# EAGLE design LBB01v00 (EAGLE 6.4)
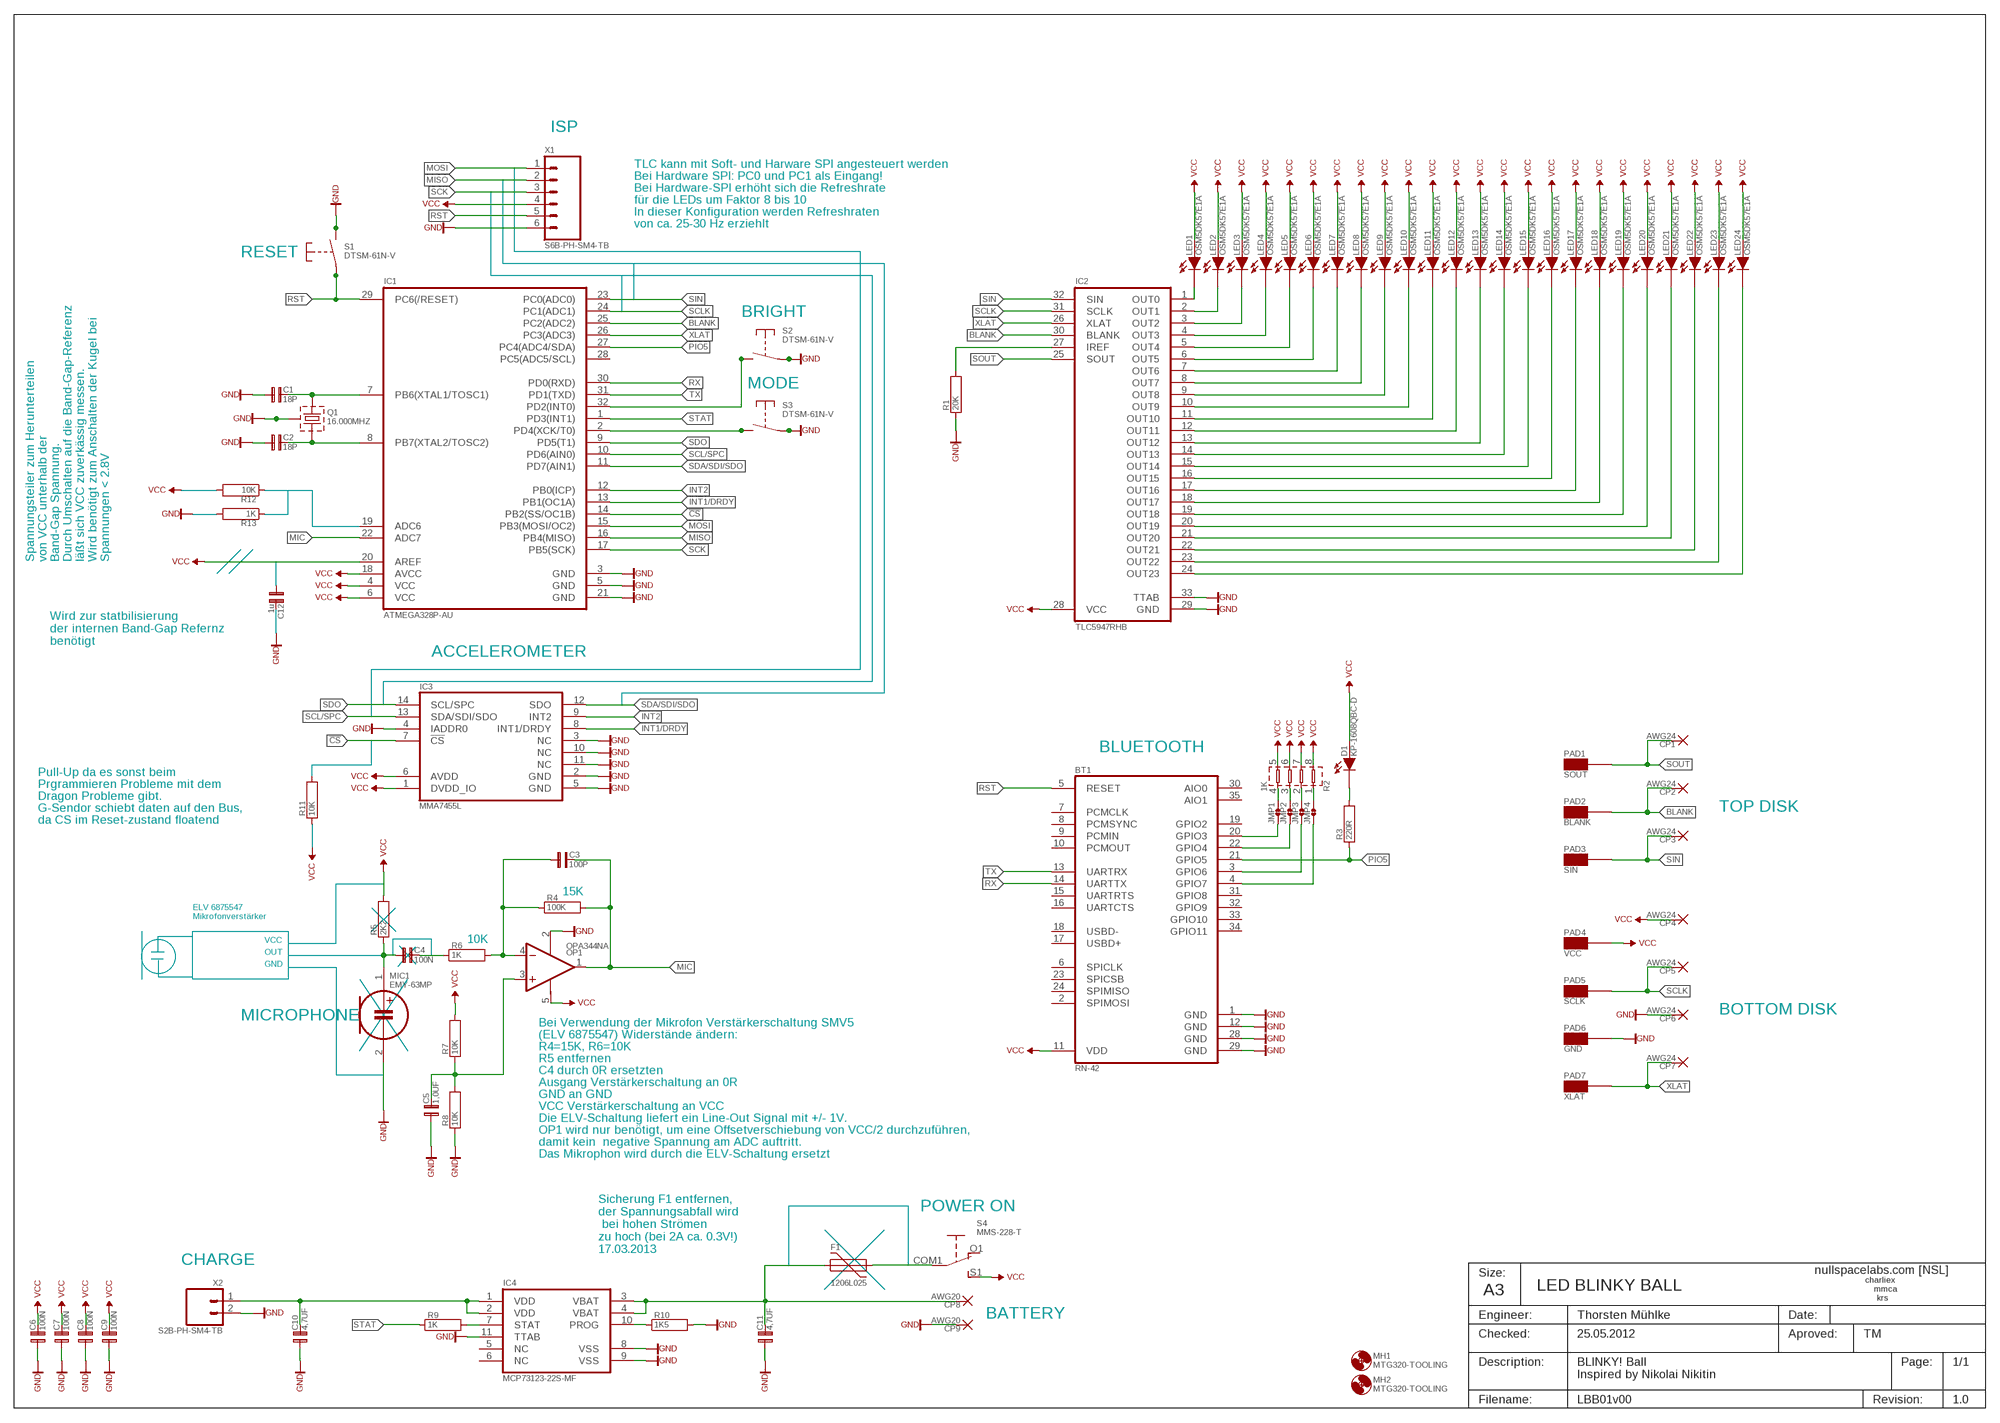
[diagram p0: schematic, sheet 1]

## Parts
BT1  RN-42  [RN-42]
C1  18P  [CAPC2012X135N]
C2  18P  [CAPC2012X135N]
C3  100P  [CAPC2012X135N]
C4  100N  [CAPC2012X135N]
C5  1,0UF  [CAPC2012X125N]
C6  100N  [CAPC2012X135N]
C7  100N  [CAPC2012X135N]
C8  100N  [CAPC2012X135N]
C9  100N  [CAPC2012X135N]
C10  4,7UF  [CAPC2012X125N]
C11  4,7UF  [CAPC2012X125N]
C12  1u  18P  [CAPC2012X135N]
CP1  AWG24  [PAD51P]
CP2  AWG24  [PAD51P]
CP3  AWG24  [PAD51P]
CP4  AWG24  [PAD51P]
CP5  AWG24  [PAD51P]
CP6  AWG24  [PAD51P]
CP7  AWG24  [PAD51P]
CP8  AWG20  [PAD81P]
CP9  AWG20  [PAD81P]
D1  KP-1608QBC-D  [LED-KP-1608QBC-D]
F1  1206L025  [FUSE-RESC3216X100N]
IC1  ATMEGA328P-AU  [QFP80P900X900X120-32N]
IC2  TLC5947RHB  [QFN50P500X500X90-33AN]
IC3  MMA7455L  [LGA-14]
IC4  MCP73123-22S-MF  [SON50P300X300X100-11N]
JMP1  SINGLE-JMP  [SINGLE-JMP]
JMP2  SINGLE-JMP  [SINGLE-JMP]
JMP3  SINGLE-JMP  [SINGLE-JMP]
JMP4  SINGLE-JMP  [SINGLE-JMP]
LED1  OSM5DK57E1A  [OSM5DK57E1A]
LED2  OSM5DK57E1A  [OSM5DK57E1A]
LED3  OSM5DK57E1A  [OSM5DK57E1A]
LED4  OSM5DK57E1A  [OSM5DK57E1A]
LED5  OSM5DK57E1A  [OSM5DK57E1A]
LED6  OSM5DK57E1A  [OSM5DK57E1A]
LED7  OSM5DK57E1A  [OSM5DK57E1A]
LED8  OSM5DK57E1A  [OSM5DK57E1A]
LED9  OSM5DK57E1A  [OSM5DK57E1A]
LED10  OSM5DK57E1A  [OSM5DK57E1A]
LED11  OSM5DK57E1A  [OSM5DK57E1A]
LED12  OSM5DK57E1A  [OSM5DK57E1A]
LED13  OSM5DK57E1A  [OSM5DK57E1A]
LED14  OSM5DK57E1A  [OSM5DK57E1A]
LED15  OSM5DK57E1A  [OSM5DK57E1A]
LED16  OSM5DK57E1A  [OSM5DK57E1A]
LED17  OSM5DK57E1A  [OSM5DK57E1A]
LED18  OSM5DK57E1A  [OSM5DK57E1A]
LED19  OSM5DK57E1A  [OSM5DK57E1A]
LED20  OSM5DK57E1A  [OSM5DK57E1A]
LED21  OSM5DK57E1A  [OSM5DK57E1A]
LED22  OSM5DK57E1A  [OSM5DK57E1A]
LED23  OSM5DK57E1A  [OSM5DK57E1A]
LED24  OSM5DK57E1A  [OSM5DK57E1A]
MH1  MTG320-TOOLING  [MTG320-TOOLING]
MH2  MTG320-TOOLING  [MTG320-TOOLING]
MIC1  EMY-63MP  [MIC-EMY-63MP]
OP1  OPA344NA  [SOT95P284X125-5N]
PAD1  SOUT  1X2  [TP_100X200]
PAD2  BLANK  1X2  [TP_100X200]
PAD3  SIN  1X2  [TP_100X200]
PAD4  VCC  1X2  [TP_100X200]
PAD5  SCLK  1X2  [TP_100X200]
PAD6  GND  1X2  [TP_100X200]
PAD7  XLAT  1X2  [TP_100X200]
Q1  16.000MHZ  [OSCCC500X700X130-4N]
R1  20K  [RESC2012X50N]
R2  1K  [RESCAXS80P160X320X50-8N]
R3  220R  [RESC2012X50N]
R4  100K  [RESC2012X50N]
R5  2K2  [RESC2012X50N]
R6  1K  [RESC2012X50N]
R7  10K  [RESC2012X50N]
R8  10K  [RESC2012X50N]
R9  1K  [RESC2012X50N]
R10  1K5  [RESC2012X50N]
R11  10K  [RESC2012X50N]
R12  10K  [RESC2012X50N]
R13  1K  10K  [RESC2012X50N]
S1  DTSM-61N-V  [SW-DTSM-61N-V]
S2  DTSM-61N-V  [SW-DTSM-61N-V]
S3  DTSM-61N-V  [SW-DTSM-61N-V]
S4  MMS-228-T  [SW-MMS-228-T]
X1  S6B-PH-SM4-TB  [S6B-PH-SM4-TB]
X2  S2B-PH-SM4-TB  [S2B-PH-SM4-TB]

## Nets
!CS: IC1.14(PB2(SS/OC1B)) IC3.7(!CS)
BLANK: CP2.1(P) IC1.25(PC2(ADC2)) IC2.30(BLANK) PAD2.1
BUTTON: IC1.32(PD2(INT0)) S2.T3 S2.T4
GND: BT1.1(GND) BT1.12(GND) BT1.28(GND) BT1.29(GND) C1.1 C2.1 C5.1 C6.1 C7.1 C8.1 C9.1 C10.1 C11.1 CP6.1(P) CP9.1(P) IC1.3(GND) IC1.5(GND) IC1.21(GND) IC2.29(GND) IC2.33(TTAB) IC3.2(GND) IC3.3(NC) IC3.4(IADDR0) IC3.5(GND) IC3.10(NC) IC3.11(NC) IC4.8(VSS) IC4.9(VSS) IC4.11(TTAB) MIC1.2(-) OP1.2(V-) PAD6.1 Q1.2(C1) Q1.4(C2) R1.1 R8.1 R10.2 S1.T3 S1.T4 S2.T1 S2.T2 S3.T1 S3.T2 X1.6 X2.2
INT1/DRDY: IC1.13(PB1(OC1A)) IC3.8(INT1/DRDY)
INT2: IC1.12(PB0(ICP)) IC3.9(INT2)
MIC: C3.2 IC1.22(ADC7) OP1.1(OUT) R4.2
MISO: IC1.16(PB4(MISO)) X1.2
MOSI: IC1.15(PB3(MOSI/OC2)) X1.1
N$1: IC2.1(OUT0) LED1.C
N$2: IC2.2(OUT1) LED2.C
N$3: IC2.3(OUT2) LED3.C
N$4: IC2.4(OUT3) LED4.C
N$5: IC2.5(OUT4) LED5.C
N$6: IC2.6(OUT5) LED6.C
N$7: IC2.7(OUT6) LED7.C
N$8: IC2.8(OUT7) LED8.C
N$9: IC2.9(OUT8) LED9.C
N$10: IC2.10(OUT9) LED10.C
N$11: IC2.11(OUT10) LED11.C
N$12: IC2.12(OUT11) LED12.C
N$13: IC2.13(OUT12) LED13.C
N$14: IC2.14(OUT13) LED14.C
N$15: IC2.15(OUT14) LED15.C
N$16: IC2.16(OUT15) LED16.C
N$17: IC2.17(OUT16) LED17.C
N$18: IC2.18(OUT17) LED18.C
N$19: IC2.19(OUT18) LED19.C
N$20: IC2.20(OUT19) LED20.C
N$21: IC2.21(OUT20) LED21.C
N$22: IC2.22(OUT21) LED22.C
N$23: IC2.23(OUT22) LED23.C
N$24: IC2.24(OUT23) LED24.C
N$25: IC2.27(IREF) R1.2
N$26: C1.2 IC1.7(PB6(XTAL1/TOSC1)) Q1.3
N$27: C2.2 IC1.8(PB7(XTAL2/TOSC2)) Q1.1
N$28: BT1.20(GPIO3) JMP1.1
N$29: BT1.22(GPIO4) JMP2.1
N$30: BT1.3(GPIO6) JMP3.1
N$31: BT1.4(GPIO7) JMP4.1
N$32: C10.2 IC4.1(VDD) IC4.2(VDD) X2.1
N$33: IC4.7(STAT) R9.2
N$34: IC4.10(PROG) R10.1
N$35: C11.2 CP8.1(P) F1.1 IC4.3(VBAT) IC4.4(VBAT)
N$36: JMP1.2 R2.4
N$37: C3.1 OP1.4(-IN) R4.1 R6.2
N$38: C4.2 R6.1
N$39: C4.1 MIC1.1(+) R5.1
N$40: C5.2 OP1.3(+IN) R7.1 R8.2
N$41: JMP2.2 R2.3
N$42: JMP4.2 R2.1
N$43: JMP3.2 R2.2
N$44: D1.C R3.2
N$45: F1.2 S4.COM1(A:P)
N$46: IC1.2(PD4(XCK/T0)) S3.T3 S3.T4
PIO5: BT1.21(GPIO5) IC1.27(PC4(ADC4/SDA)) R3.1
RST: BT1.5(RESET) IC1.29(PC6(/RESET)) S1.T1 S1.T2 X1.5
RX: BT1.14(UARTTX) IC1.30(PD0(RXD))
SCK: IC1.17(PB5(SCK)) X1.3
SCL/SPC: IC1.10(PD6(AIN0)) IC3.13(SDA/SDI/SDO)
SCLK: CP5.1(P) IC1.24(PC1(ADC1)) IC2.31(SCLK) PAD5.1
SDA/SDI/SDO: IC1.11(PD7(AIN1)) IC3.12(SDO)
SDO: IC1.9(PD5(T1)) IC3.14(SCL/SPC)
SIN: CP3.1(P) IC1.23(PC0(ADC0)) IC2.32(SIN) PAD3.1
SOUT: CP1.1(P) IC2.25(SOUT) PAD1.1
STAT: IC1.1(PD3(INT1)) R9.1
TX: BT1.13(UARTRX) IC1.31(PD1(TXD))
VCC: BT1.11(VDD) C6.2 C7.2 C8.2 C9.2 CP4.1(P) D1.A IC1.4(VCC) IC1.6(VCC) IC1.18(AVCC) IC1.20(AREF) IC2.28(VCC) IC3.1(DVDD_IO) IC3.6(AVDD) LED1.A LED2.A LED3.A LED4.A LED5.A LED6.A LED7.A LED8.A LED9.A LED10.A LED11.A LED12.A LED13.A LED14.A LED15.A LED16.A LED17.A LED18.A LED19.A LED20.A LED21.A LED22.A LED23.A LED24.A OP1.5(V+) PAD4.1 R2.5 R2.6 R2.7 R2.8 R5.2 R7.2 S4.S1(A:S) X1.4
XLAT: CP7.1(P) IC1.26(PC3(ADC3)) IC2.26(XLAT) PAD7.1
Unconnected: BT1.2(SPIMOSI) BT1.6(SPICLK) BT1.7(PCMCLK) BT1.8(PCMSYNC) BT1.9(PCMIN) BT1.10(PCMOUT) BT1.15(UARTRTS) BT1.16(UARTCTS) BT1.17(USBD+) BT1.18(USBD-) BT1.19(GPIO2) BT1.23(SPICSB) BT1.24(SPIMISO) BT1.30(AIO0) BT1.31(GPIO8) BT1.32(GPIO9) BT1.33(GPIO10) BT1.34(GPIO11) BT1.35(AIO1) C12.1 C12.2 IC1.19(ADC6) IC1.28(PC5(ADC5/SCL)) IC4.5(NC) IC4.6(NC) R11.1 R11.2 R12.1 R12.2 R13.1 R13.2 S4.COM2(B:P) S4.O1(A:O) S4.O2(B:O) S4.S2(B:S)

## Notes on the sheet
- ISP
- TLC kann mit Soft- und Harware SPI angesteuert werden
- Bei Hardware SPI: PC0 und PC1 als Eingang!
- Bei Hardware-SPI erhöht sich die Refreshrate
- für die LEDs um Faktor 8 bis 10
- In dieser Konfiguration werden Refreshraten
- von ca. 25-30 Hz erziehlt
- RESET
- BRIGHT
- MODE
- Spannungsteiler zum Herunterteilen
  von VCC unterhalb der 
  Band-Gap Spannung.
  Durch Umschalten auf die Band-Gap-Referenz
  läßt sich VCC zuverkässig messen.
  Wird benötigt zum Anschalten der Kugel bei
  Spannungen < 2.8V
- Wird zur statbilisierung 
  der internen Band-Gap Refernz 
  benötigt
- ACCELEROMETER
- BLUETOOTH
- Pull-Up da es sonst beim
- Prgrammieren Probleme mit dem
- Dragon Probleme gibt.
- G-Sendor schiebt daten auf den Bus, | TOP DISK
- da CS im Reset-zustand floatend
- 15K
- ELV 6875547
  Mikrofonverstärker
- VCC | 10K
- OUT
- GND
- BOTTOM DISK
- MICROPHONE
- Bei Verwendung der Mikrofon Verstärkerschaltung SMV5
- (ELV 6875547) Widerstände ändern:
- R4=15K, R6=10K
- R5 entfernen
- C4 durch 0R ersetzten
- Ausgang Verstärkerschaltung an 0R
- GND an GND
- VCC Verstärkerschaltung an VCC
- Die ELV-Schaltung liefert ein Line-Out Signal mit +/- 1V.
- OP1 wird nur benötigt, um eine Offsetverschiebung von VCC/2 durchzuführen,
- damit kein  negative Spannung am ADC auftritt.
- Das Mikrophon wird durch die ELV-Schaltung ersetzt
- POWER ON
- Sicherung F1 entfernen,
  der Spannungsabfall wird
   bei hohen Strömen
  zu hoch (bei 2A ca. 0.3V!)
  17.03.2013
- CHARGE
- Size: | nullspacelabs.com [NSL]
- charliex
- A3 | LED BLINKY BALL | mmca
- krs
- BATTERY | Engineer: | Thorsten Mühlke | Date:
- Checked: | 25.05.2012 | Aproved: | TM
- Description: | BLINKY! Ball | Page:
- Inspired by Nikolai Nikitin
- Filename: | Revision: | 1.0

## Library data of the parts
BT1 = Converter Roving Networks:RN-42: RN-42 Class 2 Bluetooth Module, order code: RN-42 Datasheet SolidWorks http://www.rovingnetworks.com
C1 C2 C12 = Capacitor Yageo CC0805 NP0 5pph 50V:18P: Multilayer Ceramic Capacitor 0805, NP0, 5%, 50V, order code: CC0805J*NP09BN180
C3 = Capacitor Yageo CC0805 NP0 5pph 50V:100P: Multilayer Ceramic Capacitor 0805, NP0, 5%, 50V, order code: CC0805J*NP09BN101
C4 C6-C9 = Capacitor Yageo 0805 Class2 X7R 5pph 50V:100N: Multilayer Ceramic Capacitor 0805, X7R, 5%, 50V, order code: 08052R104J9B
C5 = Capacitor Taiyo Yuden Typ 212 25V 10pph:1,0UF: High Value Multilayer Ceramic Capacitor, 1,0µF, 25V, +/-10%, order code: TMK212BJ105KG
C10 C11 = Capacitor Taiyo Yuden Typ 212 16V 10pph:4,7UF: High Value Multilayer Ceramic Capacitor, 4,7µF, 16V, +/-10%, order code: EMK212BJ475KG
CP1-CP7 = PTH-Wire:AWG24: Wire,24 guage;0.511mm diameter
CP8 CP9 = PTH-Wire:AWG20: Wire,20 guage;0.810mm diameter
D1 = Light Emitting Diode Kingbright SMD:KP-1608QBC-D: 470nm, Blue, Clear Typ, Landpattern LEDC1608X100N, order code: KP-1608QBC-D
F1 = Fuse Littlefuse 1206L:1206L025: Polyfuse I-hold=0,250A; I-trip=0,50A; 16V, order code: 1206L025
IC1 = Microcontroller Atmel:ATMEGA328P-AU: 8-Bit Microcontroller With 32kB In-System Programmable Flash, order code: ATmega328P-PU Datasheet SolidWorks http://www.atmel.com
IC2 = Linear Texas Instruments:TLC5947RHB: 24-Channel, 12-Bit PWM LED Driver with Internal Oscillator, order code: TLC5947RHB Datasheet SolidWorks http://www.ti.com
IC3 = Linear Freescale Semiconductor:MMA7455L: ±2g/±4g/±8g Three Axis Low-g Digital Output Accelerometer, order code: MMA7455L Datasheet SolidWorks http://www.freescale.com
IC4 = Regulator Microchip:MCP73123-22S-MF: Lithium Iron Phosphate (LiFePO4) Battery Charge Management Controller with Input Overvoltage Protection, order code: MCP73123-22S/MF Datasheet SolidWorks http://www.microchip.com
JMP1-JMP4 = SMT Jumper Link -0R:SINGLE-JMP: SMT 0R Solder Jumper
LED1-LED24 = Light Emitting Diode OptoSupply:OSM5DK57E1A: 5mm Flat Warm White LED, order code: OSM5DK57E1A
MH1 MH2 = Non-Plated Through Mounting Holes for Metric Based Hardware:MTG320-TOOLING: Standard Tooling Hole
MIC1 = Buzzer Ekulit:EMY-63MP: Elektret Microphone 1,5V...10V, order code: EMY-63M/P
OP1 = Linear Texas Instruments:OPA344NA: Low Power, Single-Supply, Rail to Rail Operational Amplifier, order code: OPA344NA Datasheet SolidWorks http://www.ti.com
PAD1-PAD7 = Pad Surface Mount:1X2: SMT-Pad 1,0mm x 2,0mm
Q1 = Crystal Abracon Corporation ABMM:16.000MHZ: 16.000MHz Ceramic SMD Microprocessor Crystal 7.0 x 5.0 x 1.3mm, order code: ABMM-16.000MHZ-B2-T Datasheet SolidWorks http://www.abracon.com
R1 = Resistor Yageo RC0805 1pph:20K: Chip resistor RC0805, 1%, order code: RC0805FR-0720K
R2 = Resistor Bourns CAY16 5pph 4 Isolated:1K: Chip Resistor Array CAY16, 5%, 4 Isolated Resistors, Convex, order code: CAY16-102J4 Datasheet SolidWorks http://www.bourns.com
R3 = Resistor Yageo RC0805 1pph:220R: Chip resistor RC0805, 1%, order code: RC0805FR-07220R
R4 = Resistor Yageo RC0805 1pph:100K: Chip resistor RC0805, 1%, order code: RC0805FR-07100K
R5 = Resistor Yageo RC0805 1pph:2K2: Chip resistor RC0805, 1%, order code: RC0805FR-072K2
R6 R9 = Resistor Yageo RC0805 1pph:1K: Chip resistor RC0805, 1%, order code: RC0805FR-071K
R7 R8 R11-R13 = Resistor Yageo RC0805 1pph:10K: Chip resistor RC0805, 1%, order code: RC0805FR-0710K
R10 = Resistor Yageo RC0805 1pph:1K5: Chip resistor RC0805, 1%, order code: RC0805FR-071K5
S1-S3 = Switch Diptronics:DTSM-61N-V: Tact Switch, h = 4,3 mm, order code: DTSM-61N-V Datasheet SolidWorks http://www.dip.com.tw
S4 = Switch Knitter:MMS-228-T: Microminiature Slide Switches, (ON - ON), order code: MMS_228-T Datasheet SolidWorks http://www.knitter-switch.com
X1 = Connector JST PH-SM4:S6B-PH-SM4-TB: Disconnectable Crimp style connector, Typ SM4, 06pol, Side entry type, order code: S6B-PH-SM4-TB Datasheet SolidWorks http://www.jst.de
X2 = Connector JST PH-SM4:S2B-PH-SM4-TB: Disconnectable Crimp style connector, Typ SM4, 02pol, Side entry type, order code: S2B-PH-SM4-TB

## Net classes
0 default: width 0.2 mm, drill 0.3 mm, clearance 0.2 mm

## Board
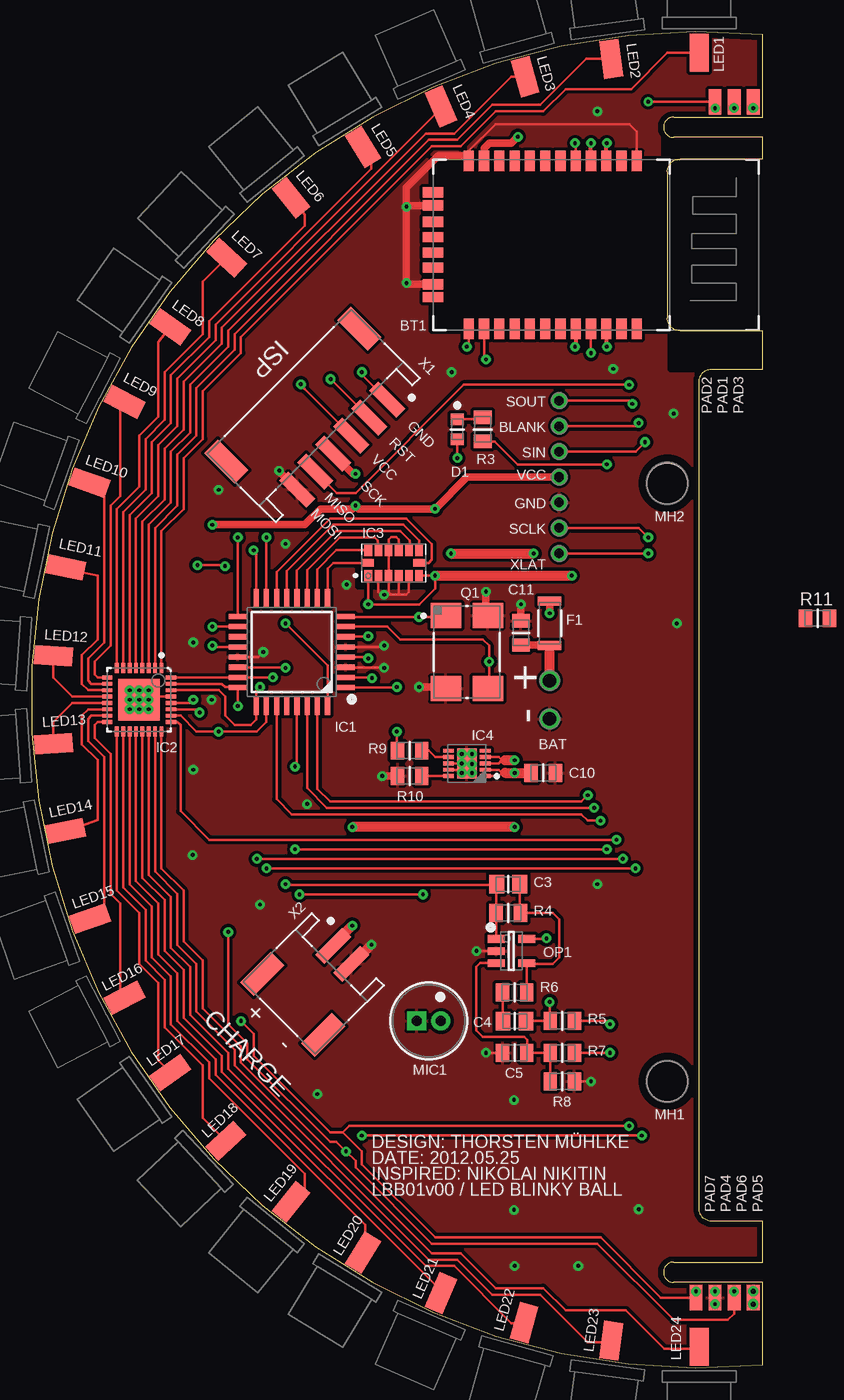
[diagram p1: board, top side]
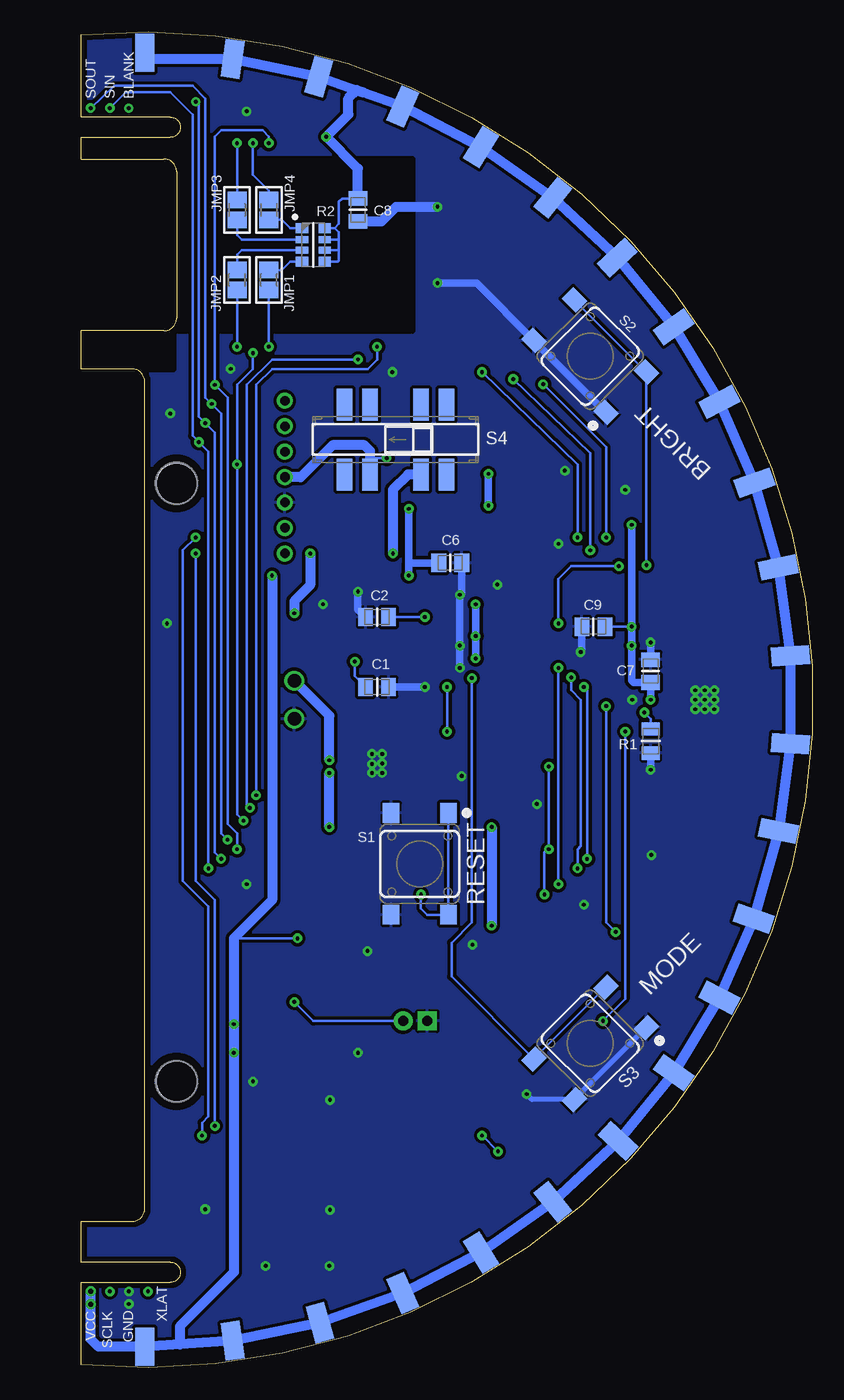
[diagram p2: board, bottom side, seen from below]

Size 57.43 x 105 mm. Coordinates in mm from the lower left corner, seen from the top.
Outline: 57.43,96.7 50.43,96.7 arc-180 50.43,98.3 57.43,98.3 57.43,104.76 arc191 57.43,0.24 57.43,6.7 50.43,6.7 arc-180 50.43,8.3 57.43,8.3 57.43,11.5 53.43,11.5 arc-90 52.43,12.5 52.43,77.5 arc-90 53.43,78.5 57.43,78.5 57.43,81.5 50.93,81.5 arc-90 49.93,82.5 49.93,94 arc-90 50.93,95 57.43,95 57.43,96.7
Copper layers (1*16): Top 0.018mm / dielectric 1.55mm / Bottom 0.018mm
Design rules "default": minimum track width 0.15mm, minimum drill 0.25mm, track to track 0.15mm, track to pad 0.15mm, pad to pad 0.15mm, via to via 0.15mm, smd to smd 0.15mm, copper to edge 0.45mm, drill to drill 0.3mm, minimum pad ring 0.2mm, minimum via ring 0.2mm, stop-mask expansion 0.1mm, vias tented up to drill 0mil, thermal gap 0.2mm
tRestrict: area 31.4,81.5 to 50.2,95; area 49.7,95 to 57.4,96.7; area 50.2,78.5 to 57.4,81.5; area 32.3,46.8 to 32.8,47.7; area 6.6,50.7 to 10.2,54.3; area 11.3,52.6 to 11.5,52.9; area 27,62.2 to 29.8,63.8; area 27.4,64.1 to 29.1,65.4; area 33.2,47.2 to 33.5,47.8; area 26.8,61.4 to 30.9,61.7; area 25.6,61.4 to 26.1,62.9; area 53,4.1 to 54.3,4.5
bRestrict: area 31.4,81.5 to 50.2,95; area 49.7,95 to 57.4,96.7; area 50.2,78.5 to 57.4,81.5

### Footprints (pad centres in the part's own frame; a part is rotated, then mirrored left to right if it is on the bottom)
RN-42 = smd 0.8 x 1.6: 1 -6.6,-6.6; 2 -5.4,-6.6; 3 -4.2,-6.6; 4 -3,-6.6; 5 -1.8,-6.6; 6 -0.6,-6.6; 7 0.6,-6.6; 8 1.8,-6.6; 9 3,-6.6; 10 4.2,-6.6; 11 5.4,-6.6; 12 6.6,-6.6; 13 6.6,6.6; 14 5.4,6.6; 15 4.2,6.6; 16 3,6.6; 17 1.8,6.6; 18 0.6,6.6; 19 -0.6,6.6; 20 -1.8,6.6; 21 -3,6.6; 22 -4.2,6.6; 23 -5.4,6.6; 24 -6.6,6.6 | smd 1.6 x 0.8: 28 9.4,3.1; 29 9.4,-3.1; 30 9.4,4.1; 31 9.4,1.8; 32 9.4,0.6; 33 9.4,-0.6; 34 9.4,-1.8; 35 9.4,-4.122
CAPC2012X135N = smd 1.15 x 1.45: 1 -0.9,0; 2 0.9,0
CAPC2012X125N = smd 1.05 x 1.4: 1 -0.95,0; 2 0.95,0
PAD51P = drill 0.75 pad 1.25: 1 0,0
PAD81P = drill 1.05 pad 1.55: 1 0,0
LED-KP-1608QBC-D = smd 0.9 x 1: A 0.8,0; C -0.8,0
FUSE-RESC3216X100N = smd 0.7 x 1.85: 1 -1.75,0; 2 1.75,0
QFP80P900X900X120-32N = smd 1.4 x 0.4: 1 -4.25,2.8; 2 -4.25,2; 3 -4.25,1.2; 4 -4.25,0.4; 5 -4.25,-0.4; 6 -4.25,-1.2; 7 -4.25,-2; 8 -4.25,-2.8; 17 4.25,-2.8; 18 4.25,-2; 19 4.25,-1.2; 20 4.25,-0.4; 21 4.25,0.4; 22 4.25,1.2; 23 4.25,2; 24 4.25,2.8 | smd 0.4 x 1.4: 9 -2.8,-4.25; 10 -2,-4.25; 11 -1.2,-4.25; 12 -0.4,-4.25; 13 0.4,-4.25; 14 1.2,-4.25; 15 2,-4.25; 16 2.8,-4.25; 25 2.8,4.25; 26 2,4.25; 27 1.2,4.25; 28 0.4,4.25; 29 -0.4,4.25; 30 -1.2,4.25; 31 -2,4.25; 32 -2.8,4.25
QFN50P500X500X90-33AN = smd 0.8 x 0.3: 1 -2.5,1.75; 2 -2.5,1.25; 3 -2.5,0.75; 4 -2.5,0.25; 5 -2.5,-0.25; 6 -2.5,-0.75; 7 -2.5,-1.25; 8 -2.5,-1.75; 17 2.5,-1.75; 18 2.5,-1.25; 19 2.5,-0.75; 20 2.5,-0.25; 21 2.5,0.25; 22 2.5,0.75; 23 2.5,1.25; 24 2.5,1.75 | smd 0.3 x 0.8: 9 -1.75,-2.5; 10 -1.25,-2.5; 11 -0.75,-2.5; 12 -0.25,-2.5; 13 0.25,-2.5; 14 0.75,-2.5; 15 1.25,-2.5; 16 1.75,-2.5; 25 1.75,2.5; 26 1.25,2.5; 27 0.75,2.5; 28 0.25,2.5; 29 -0.25,2.5; 30 -0.75,2.5; 31 -1.25,2.5; 32 -1.75,2.5 | smd 3.25 x 3.25: 33 0,0
LGA-14 = smd 0.6 x 0.9: 1 -2,-1; 2 -1.2,-1; 3 -0.4,-1; 4 0.4,-1; 5 1.2,-1; 6 2,-1; 8 2,1; 9 1.2,1; 10 0.4,1; 11 -0.4,1; 12 -1.2,1; 13 -2,1 | smd 0.9 x 0.6: 7 2,0; 14 -2,0
SON50P300X300X100-11N = smd 0.85 x 0.3: 1 -1.45,1; 2 -1.45,0.5; 3 -1.45,0; 4 -1.45,-0.5; 5 -1.45,-1; 6 1.45,-1; 7 1.45,-0.5; 8 1.45,0; 9 1.45,0.5; 10 1.45,1 | smd 1.55 x 2.35: 11 0,0
SINGLE-JMP = smd 1.5 x 1.3: 1 0,0.8; 2 0,-0.8
OSM5DK57E1A = smd 3 x 1.5 bottom: A 1.9,0 | smd 3 x 1.5: C 1.9,0
MTG320-TOOLING = hole 3.2: 0,0
MIC-EMY-63MP = drill 0.8 pad 1.5: 1 0.95,0 | drill 0.8 pad 1.5 square: 2 -0.95,0
SOT95P284X125-5N = smd 1.35 x 0.6: 1 -1.2,0.95; 2 -1.2,0; 3 -1.2,-0.95; 4 1.2,-0.95; 5 1.2,0.95
TP_100X200 = smd 1 x 2: 1 0,0
OSCCC500X700X130-4N = smd 2.4 x 1.95: 1 -1.65,2.874; 2 -1.65,-2.876; 3 1.65,-2.876; 4 1.65,2.874
RESC2012X50N = smd 1.05 x 1.4: 1 -0.95,0; 2 0.95,0
RESCAXS80P160X320X50-8N = smd 0.95 x 0.8: 1 -0.9,1.325; 4 -0.9,-1.325; 5 0.9,-1.325; 8 0.9,1.325 | smd 0.95 x 0.55: 2 -0.9,0.4; 3 -0.9,-0.4; 6 0.9,-0.4; 7 0.9,0.4
SW-DTSM-61N-V = smd 1.55 x 1.3: T1 -4,2.25; T2 4,2.25; T3 -4,-2.25; T4 4,-2.25
SW-MMS-228-T = smd 1.2 x 2.5: COM1 -2,2.75; COM2 -2,-2.75; NC1 4,2.75; NC2 4,-2.75; O1 -4,2.75; O2 -4,-2.75; S1 2,2.75; S2 2,-2.75
S6B-PH-SM4-TB = smd 1 x 3: 1 5,-7; 2 3,-7; 3 1,-7; 4 -1,-7; 5 -3,-7; 6 -5,-7 | smd 1.5 x 3.4: P$3 -7.4,-1.5; P$4 7.4,-1.5
S2B-PH-SM4-TB = smd 1 x 3: 1 1,-7; 2 -1,-7 | smd 1.5 x 3.4: P$3 -3.4,-1.5; P$4 3.4,-1.5

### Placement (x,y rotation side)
BT1  40.93,88.25 180 top
C1  34.18,53.5 180 bottom
C2  34.18,59 0 bottom
C3  37.43,38 180 top
C4  37.93,27.25 180 top
C5  37.93,24.75 0 top
C6  28.43,63.25 180 bottom
C7  12.68,54.75 270 bottom
C8  35.68,91 90 bottom
C9  17.18,58.25 0 bottom
C10  40.18,46.75 180 top
C11  38.43,57.75 270 top
C12  not placed on the board
CP1  41.43,76 0 top
CP2  41.43,74 0 top
CP3  41.43,72 0 top
CP4  41.43,70 0 top
CP5  41.43,66 0 top
CP6  41.43,68 0 top
CP7  41.43,64 0 top
CP8  40.68,54 0 top
CP9  40.68,51 0 top
D1  33.43,73.75 270 top
F1  40.68,58.5 90 top
IC1  20.43,56.25 180 top
IC2  8.43,52.5 270 top
IC3  28.43,63.25 0 top
IC4  34.18,47.5 180 top
JMP1  42.68,85.5 180 bottom
JMP2  45.18,85.5 180 bottom
JMP3  45.18,91 0 bottom
JMP4  42.68,91 0 bottom
LED1  52.43,105.25 270 top
LED2  45.27,104.76 277.8 top
LED3  38.25,103.31 285.6 top
LED4  31.4,100.87 293.5 top
LED5  25.03,97.57 301.3 top
LED6  19.16,93.44 309.1 top
LED7  13.92,88.54 316.9 top
LED8  9.33,82.91 324.8 top
LED9  5.6,76.77 332.6 top
LED10  2.74,70.19 340.4 top
LED11  0.8,63.29 348.2 top
LED12  -0.19,56.09 356.1 top
LED13  -0.19,48.91 3.9 top
LED14  0.78,41.8 11.7 top
LED15  2.79,34.66 19.5 top
LED16  5.6,28.22 27.4 top
LED17  9.33,22.09 35.2 top
LED18  13.85,16.52 43 top
LED19  19.16,11.56 50.9 top
LED20  25.03,7.43 58.7 top
LED21  31.4,4.12 66.5 top
LED22  38.16,1.72 74.3 top
LED23  45.27,0.24 82.2 top
LED24  52.43,-0.25 90 top
MH1  49.93,22.5 180 top
MH2  49.93,69.5 180 top
MIC1  31.18,27.25 0 top
OP1  37.68,32.75 0 top
PAD1  56.68,99.5 0 top
PAD2  53.68,99.5 0 top
PAD3  55.18,99.5 0 top
PAD4  56.68,5.5 0 top
PAD5  55.18,5.5 0 top
PAD6  53.68,5.5 0 top
PAD7  52.18,5.5 0 top
Q1  34.18,56.25 0 top
R1  12.68,49.25 90 bottom
R2  39.18,88.25 0 bottom
R3  35.43,73.75 90 top
R4  37.43,35.75 180 top
R5  41.68,27.25 0 top
R6  37.93,29.5 0 top
R7  41.68,24.75 0 top
R8  41.68,22.5 180 top
R9  29.68,48.5 0 top
R10  29.68,46.5 180 top
R11  not placed on the board
R12  not placed on the board
R13  not placed on the board
S1  30.83,39.6 270 bottom
S2  17.43,79.5 135 bottom
S3  17.43,25.5 225 bottom
S4  32.73,72.95 180 bottom
X1  19.43,77.5 45 top
X2  19.43,27.5 135 top

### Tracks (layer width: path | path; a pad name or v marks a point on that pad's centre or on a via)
!CS
  Top 0.2: IC1.14 19.23,62.55 23.43,66.75 29.43,66.75 31.43,64.75 31.43,63.5 31.18,63.25 IC3.7
BLANK  (via drill 0.3 pad 0.7, 0.3 pad 0.75)
  Top 0.2: IC2.30 14.68,53.25 15.18,52.75 15.18,51.25 15.93,50.5 17.18,50.5 17.63,50.95 IC1.25 17.63,53.2 v17.93,53.5 | v46.43,40 v17.68,40 | v48.43,99.5 53.43,99.5 53.68,99.25 v53.68,99 PAD2.1 | CP2.1 47.43,74 v47.68,74.25
  Bottom 0.2: v48.43,99.5 48.18,99.25 48.18,74.75 v47.68,74.25 46.93,73.5 46.93,40.5 v46.43,40 | v17.93,53.5 17.68,53.25 v17.68,40
BUTTON  (via drill 0.3 pad 0.75)
  Top 0.2: IC1.32 23.23,55.2 v19.93,58.5 | v13.01,63.08 15.1,63.08 v15.18,63
  Bottom 0.2: S2.T4 S2.T3 v13.01,63.08 | v19.93,58.5 19.93,62 18.93,63 v15.18,63
GND  (via drill 0.3 pad 0.75)
  Top 0.2: 29.68,62.2 IC3.5 29.63,60.95 29.43,60.75 28.93,60.75 | IC2.29 9.18,52.75 v9.18,52.5 | BT1.1 47.53,97.15 46.93,97.75 36.43,97.75 34.33,95.65 BT1.12 34.18,95.25 | R8.1 v43.93,22.5 | v35.68,24.75 C5.1 | OP1.2 v34.93,32.75 | IC1.21 17.78,55.85 v18.18,56.25 | IC1.3 27.38,55.05 v27.68,55 | IC1.5 27.58,56.65 v27.68,56.75 | IC3.2 27.23,60.95 27.43,60.75 v27.68,60.75 28.18,60.75 | 28.93,60.75 28.18,60.75 | IC3.4 28.83,60.85 28.93,60.75 | 28.18,60.75 28.03,60.9 IC3.3 IC3.11 28.03,65.1 28.23,65.3 28.63,65.3 28.83,65.1 IC3.10 | IC4.8 v33.78,47.5 | IC4.9 33.78,47 v33.78,46.75
  Top 0.6: BT1.29 29.58,91.35 v29.43,91.25 | v29.43,91.25 29.43,92.75 31.93,95.25 34.18,95.25 | BT1.28 29.53,85.15 v29.43,85.25 v29.43,91.25 | Q1.4 35.68,59.27 v35.68,61 | Q1.2 32.41,53.5 v30.43,53.5 | C11.1 v38.43,60 | R10.2 v27.53,46.5 | X1.6 19.43,70.43 v19.43,70.5
  Top 0.8: X2.2 25.18,31.74 v26.68,33.25
  Bottom 0.406: S3.T1 S3.T2 22.01,21.08 v22.43,21.5
  Bottom 0.6: C6.1 27.53,60.85 v27.68,60.75 v27.68,56.75 v27.68,55 | C7.1 v12.68,57 | R1.1 v12.68,47 | C9.1 18.08,56.35 v18.18,56.25 | S2.T1 S2.T2 26.37,85.25 v29.43,85.25 | C2.1 35.68,59.6 v35.68,61 | C1.1 v30.43,53.5
  Bottom 0.8: C8.1 33.83,90.1 32.68,91.25 v29.43,91.25
  other vias: 8.43,52.5 7.68,52.5 7.68,53.25 8.43,53.25 9.18,53.25 9.18,51.75 8.43,51.75 7.68,51.75 33.78,48.25 44.43,38 53.68,6 50.68,58.5 50.43,75 45.68,78.5 44.43,98.75 17.93,36.4 42.93,8 12.63,40.3 37.88,21.05 37.88,12.4 37.93,8 47.68,12.45 32.98,78.25 14.68,69 14.13,52.5 19.93,64.75 53.68,5 34.58,46.75 34.58,47.45 34.58,48.25 24.73,61.55 21.63,44.3
  pour Top (isolate 0.25): -0.57,-0.5 57.43,-0.5 57.43,105.5 -0.57,105.5
  pour Bottom (isolate 0.25): -0.57,105.5 57.43,105.5 57.43,-0.5 -0.57,-0.5
INT1/DRDY
  Top 0.2: IC1.13 20.03,62.6 23.68,66.25 29.18,66.25 30.43,65 IC3.8
INT2
  Top 0.2: IC1.12 20.83,62.65 23.93,65.75 28.93,65.75 29.68,65 29.68,64.3 IC3.9
MIC  (via drill 0.3 pad 0.75)
  Top 0.2: OP1.1 R4.2 36.48,37.95 | 36.48,37.95 C3.2 | 36.48,37.95 20.23,37.95 v19.93,38 | IC1.22 19.88,55.05 v19.93,55
  Bottom 0.2: v19.93,38 v19.93,55
MISO  (via drill 0.3 pad 0.75)
  Top 0.2: IC1.16 17.63,64.05 v17.43,64.25 | X1.2 23.68,77.49 v23.48,77.7
  Bottom 0.2: v17.43,64.25 17.43,71.9 v23.48,77.7
MOSI  (via drill 0.3 pad 0.75)
  Top 0.2: IC1.15 v18.43,65.25 | X1.1 25.93,78.07 v25.93,78.25
  Bottom 0.2: v18.43,65.25 18.43,71 v25.93,78.25
N$1
  Top 0.2: LED1.C 49.93,103.35 47.08,100.5 41.93,100.5 40.18,98.75 36.43,98.75 33.68,96 31.43,96 16.43,81 16.43,79.75 13.43,76.75 13.43,73 11.93,71.5 11.93,67.5 10.18,65.75 IC2.1
N$2
  Top 0.2: LED2.C 43.56,102.88 39.93,99.25 36.18,99.25 33.43,96.5 31.18,96.5 15.93,81.25 15.93,80 12.93,77 12.93,73.25 11.43,71.75 11.43,67.75 9.68,66 IC2.2
N$3
  Top 0.2: LED3.C 37.66,101.48 33.18,97 30.93,97 15.43,81.5 15.43,80.25 12.43,77.25 12.43,73.5 10.93,72 10.93,68 9.18,66.25 IC2.3
N$4
  Top 0.2: LED4.C 32.41,99.22 14.93,81.75 14.93,80.5 11.93,77.5 11.93,73.75 10.43,72.25 10.43,68.25 8.68,66.5 IC2.4
N$5
  Top 0.2: IC2.5 8.18,66.75 9.93,68.5 9.93,72.5 11.43,74 11.43,77.75 14.43,80.75 14.43,82 26.68,94.25 26.68,94.53 LED5.C
N$6
  Top 0.2: IC2.6 7.68,67 9.43,68.75 9.43,72.75 10.93,74.25 10.93,78 13.93,81 13.93,82.25 21.43,89.75 21.43,90.64 LED6.C
N$7
  Top 0.2: IC2.7 7.18,67.25 8.93,69 8.93,73 10.43,74.5 10.43,78.25 13.43,81.25 13.43,85.37 LED7.C
N$8
  Top 0.2: IC2.8 6.68,67.5 8.43,69.25 8.43,73.25 9.93,74.75 9.93,80.61 LED8.C
N$9
  Top 0.2: IC2.9 5.18,54.25 4.93,54.5 4.93,55.5 6.18,56.75 6.18,67.75 6.93,68.5 6.93,75.55 LED9.C
N$10
  Top 0.2: IC2.10 4.68,53.75 4.43,54 4.43,55.75 5.68,57 5.68,69.15 LED10.C
N$11
  Top 0.2: IC2.11 4.43,53.25 3.93,53.75 3.93,56 5.18,57.25 5.18,62.25 2.81,62.75 LED11.C
N$12
  Top 0.2: IC2.12 3.18,52.75 1.68,54.25 1.68,55.94 LED12.C
N$13
  Top 0.2: IC2.13 3.18,52.25 1.68,50.75 1.68,49.06 LED13.C
N$14
  Top 0.2: IC2.14 4.43,51.75 3.93,51.25 3.93,49 5.18,47.75 5.18,43.05 3.2,42.35 LED14.C
N$15
  Top 0.2: IC2.15 4.68,51.25 4.43,51 4.43,49.25 5.68,48 5.68,35.75 5.43,35.5 4.79,35.5 LED15.C
N$16
  Top 0.2: IC2.16 5.18,50.75 4.93,50.5 4.93,49.5 6.18,48.25 6.18,37.25 6.93,36.5 6.93,29.45 LED16.C
N$17
  Top 0.2: IC2.17 6.68,37.5 8.43,35.75 8.43,31.75 9.93,30.25 9.93,24.14 LED17.C
N$18
  Top 0.2: IC2.18 7.18,37.75 8.93,36 8.93,32 10.43,30.5 10.43,26.75 13.43,23.75 13.43,19.63 LED18.C
N$19
  Top 0.2: IC2.19 7.68,38 9.43,36.25 9.43,32.25 10.93,30.75 10.93,27 13.93,24 13.93,22.75 21.43,15.25 21.43,14.11 LED19.C
N$20
  Top 0.2: IC2.20 8.18,38.25 9.93,36.5 9.93,32.5 11.43,31 11.43,27.25 14.43,24.25 14.43,23 26.18,11.25 26.18,9.22 LED20.C
N$21
  Top 0.2: IC2.21 8.68,38.5 10.43,36.75 10.43,32.75 11.93,31.25 11.93,27.5 14.93,24.5 14.93,23.25 31.68,6.5 31.68,6.34 LED21.C
N$22
  Top 0.2: IC2.22 9.18,38.75 10.93,37 10.93,33 12.43,31.5 12.43,27.75 15.43,24.75 15.43,23.5 30.93,8 33.18,8 37.68,3.5 38.63,3.5 LED22.C
N$23
  Top 0.2: IC2.23 9.68,39 11.43,37.25 11.43,33.25 12.93,31.75 12.93,28 15.93,25 15.93,23.75 31.18,8.5 33.43,8.5 36.18,5.75 39.93,5.75 43.68,2 45.41,2 LED23.C
N$24
  Top 0.2: IC2.24 10.18,39.25 11.93,37.5 11.93,33.5 13.43,32 13.43,28.25 16.43,25.25 16.43,24 31.43,9 33.68,9 36.43,6.25 40.18,6.25 41.93,4.5 46.68,4.5 49.68,1.5 52.28,1.5 LED24.C
N$25  (via drill 0.3 pad 0.75)
  Top 0.2: IC2.27 12.93,51.75 v13.18,51.5
  Bottom 0.2: R1.2 12.68,51 v13.18,51.5
N$26  (via drill 0.3 pad 0.75)
  Top 0.2: IC1.7 27.93,58.25 28.93,57.25 35.43,57.25 35.93,56.75 v35.93,55.5 35.93,53.47 Q1.3
  Bottom 0.2: C1.2 35.93,54.35 v35.93,55.5
N$27  (via drill 0.3 pad 0.75)
  Top 0.2: Q1.1 32.41,59 v30.43,59 24.73,59 IC1.8
  Bottom 0.2: C2.2 v30.43,59
N$28  (via drill 0.3 pad 0.75)
  Top 0.3: BT1.20 42.73,80.3 v42.68,80.25
  Bottom 0.2: JMP1.1 v42.68,80.25
N$29  (via drill 0.3 pad 0.75)
  Top 0.3: BT1.22 45.13,80.3 v45.18,80.25
  Bottom 0.2: JMP2.1 v45.18,80.25
N$30  (via drill 0.3 pad 0.75)
  Top 0.3: BT1.3 45.13,96.2 v45.18,96.25
  Bottom 0.2: JMP3.1 v45.18,96.25
N$31  (via drill 0.3 pad 0.75)
  Top 0.3: BT1.4 v43.93,96.25
  Bottom 0.2: JMP4.1 42.68,92.5 43.93,93.75 v43.93,96.25
N$32  (via drill 0.3 pad 0.75)
  Top 0.2: IC4.2 36.68,47 36.93,46.75 | IC4.1 36.68,46.5 36.93,46.75 | 36.93,46.75 37.18,46.75
  Top 0.5: X2.1 23.75,33.16
  Top 0.8: 37.18,46.75 v37.93,46.75 C10.2 | v37.93,42.5 v25.18,42.5 | 23.75,33.16 23.75,33.31 v25.18,34.75
  Bottom 0.8: v25.18,42.5 v25.18,34.75 | v37.93,42.5 v37.93,46.75
N$33
  Top 0.2: IC4.7 31.68,48 31.18,48.5 R9.2
N$34
  Top 0.2: IC4.10 R10.1
N$35  (via drill 0.3 pad 0.75)
  Top 0.2: IC4.4 36.68,48 36.93,47.75 | IC4.3 36.68,47.5 36.93,47.75 | 36.93,47.75 37.18,47.75
  Top 0.5: 40.68,56.25 F1.1
  Top 0.6: C11.2 40.63,56.8 F1.1
  Top 0.8: 37.18,47.75 v37.93,47.75 | CP8.1 40.68,56.25
  Bottom 0.8: v37.93,47.75 37.93,51.25 CP8.1
N$36
  Bottom 0.2: R2.4 41.01,86.92 41.68,86.25 42.63,86.25 JMP1.2
N$37
  Top 0.2: R6.2 OP1.4 38.93,31.75 40.93,31.75 41.43,32.25 41.43,35.25 40.93,35.75 R4.1 38.33,35.8 C3.1
N$38
  Top 0.2: R6.1 36.98,27.3 C4.2
N$39  (via drill 0.3 pad 0.75)
  Top 0.2: C4.1 R5.1 40.68,27.3 v40.68,28.75
  Bottom 0.2: MIC1.1 39.18,27.25 v40.68,28.75
N$40
  Top 0.2: R8.2 R7.1 C5.2 38.93,24.8 38.93,25.75 38.68,26 35.43,26 34.93,26.5 34.93,31.5 35.23,31.8 OP1.3
N$41
  Bottom 0.2: R2.3 44.83,87.85 45.18,87.5 JMP2.2
N$42
  Bottom 0.2: R2.1 41.01,89.57 41.68,90.25 42.63,90.25 JMP4.2
N$43
  Bottom 0.2: R2.2 44.83,88.65 45.18,89 JMP3.2
N$44
  Top 0.2: D1.C 35.53,74.55 R3.2
N$45  (via drill 0.3 pad 0.75)
  Top 0.6: F1.2 v40.68,59.3
  Top 0.8: v32.93,64 v39.43,64
  Bottom 0.8: S4.COM1 31.73,70.2 32.93,69 v32.93,64 | v39.43,64 39.43,61.5 F1.2 v40.68,59.3
N$46  (via drill 0.3 pad 0.75)
  Top 0.2: IC1.2 26.68,54.25 v26.73,54.2
  Bottom 0.2: v26.73,54.2 26.73,35 28.33,33.4 28.33,30.74 S3.T4 S3.T3
PIO5  (via drill 0.3 pad 0.75)
  Top 0.2: BT1.21 v43.93,79.75 | v44.68,43 43.68,43 43.18,43.5 20.43,43.5 19.23,44.7 IC1.27 | R3.1 36.38,72.8 38.18,71 v45.18,71
  Bottom 0.2: v43.93,79.75 43.93,78.5 45.18,77.25 v45.18,71 45.18,43.5 v44.68,43
RST  (via drill 0.3 pad 0.75)
  Top 0.2: BT1.5 42.73,96.2 v42.68,96.25 | IC1.29 20.83,47.35 v20.68,47.25 | v20.68,40.75 v45.18,40.75 | v46.93,77.25 33.93,77.25 25.43,68.75 23.94,68.75 X1.5 | v21.03,37.2 v30.73,37.2
  Bottom 0.2: v42.68,96.25 42.68,96.75 43.18,97.25 46.43,97.25 46.93,96.75 v46.93,77.25 45.93,76.25 45.93,42.75 45.18,42 v45.18,40.75 | v20.68,47.25 v20.68,40.75 20.78,40.75 21.03,40.5 v21.03,37.2 | S1.T1 S1.T2 30.23,35.6 30.73,36.1 v30.73,37.2
RX  (via drill 0.3 pad 0.75)
  Top 0.2: BT1.14 35.53,79.35 v35.68,79.25 | v44.18,44 23.18,44 21.63,45.55 IC1.30
  Bottom 0.2: v35.68,79.25 42.43,79.25 44.43,77.25 44.43,44.25 v44.18,44
SCK  (via drill 0.3 pad 0.75)
  Top 0.2: IC1.17 v16.18,65.25 | X1.3 21.43,76.91 v21.13,77.3
  Bottom 0.2: v16.18,65.25 16.18,72.35 v21.13,77.3
SCL/SPC
  Top 0.2: IC1.10 22.43,62.75 23.93,64.25 IC3.13
SCLK  (via drill 0.3 pad 0.75)
  Top 0.2: IC2.31 14.93,53.75 15.18,53.5 16.13,53.5 IC1.24 v16.18,52 | v15.43,34.25 15.43,27 16.93,25.5 16.93,24.25 23.43,17.75 23.93,17.75 v24.68,17 25.43,16.25 25.43,15.75 31.43,9.75 44.43,9.75 50.43,3.75 54.68,3.75 55.18,4.25 PAD5.1 v55.18,6 | CP5.1 47.68,66 v48.43,65.25 | v47.93,18.25 v25.93,18.25
  Bottom 0.2: v16.18,52 16.18,35 v15.43,34.25 | v48.43,65.25 49.43,64.25 49.43,38.25 47.43,36.25 47.43,19.75 47.93,19.25 v47.93,18.25 | v25.93,18.25 v24.68,17
SDA/SDI/SDO
  Top 0.2: IC1.11 21.63,62.7 24.18,65.25 26.93,65.25 27.18,65 27.18,64.3 IC3.12
SDO
  Top 0.2: IC1.9 23.23,62.8 23.68,63.25 IC3.14
SIN  (via drill 0.3 pad 0.75)
  Top 0.2: IC2.32 IC1.23 v18.93,54.25 | v47.43,39.25 v18.43,39.25 | CP3.1 47.43,72 v48.18,72.75 | v55.18,99 PAD3.1
  Bottom 0.2: v47.43,39.25 47.43,72 v48.18,72.75 48.68,73.25 48.68,98.5 50.43,100.25 53.93,100.25 v55.18,99 | v18.93,54.25 18.93,53.25 18.18,52.5 18.18,41 18.43,40.75 v18.43,39.25
SOUT  (via drill 0.3 pad 0.75)
  Top 0.2: IC2.25 11.43,50.75 11.68,50.5 11.68,43.75 13.93,41.5 v45.93,41.5 | CP1.1 46.93,76 v47.18,75.75 | v56.68,99 PAD1.1
  Bottom 0.2: v45.93,41.5 46.43,42 46.43,75 v47.18,75.75 47.68,76.25 47.68,99.75 48.68,100.75 54.83,100.75 v56.68,99
STAT  (via drill 0.3 pad 0.75)
  Top 0.2: IC1.1 28.73,53.45 v28.68,53.5 | v28.68,50 28.68,48.55 R9.1
  Bottom 0.2: v28.68,53.5 v28.68,50
TX  (via drill 0.3 pad 0.75)
  Top 0.2: BT1.13 34.33,80.4 v34.18,80.25 | v43.68,45 43.18,44.5 23.43,44.5 22.43,45.5 IC1.31
  Bottom 0.2: v34.18,80.25 34.18,79.25 34.93,78.5 42.43,78.5 43.68,77.25 v43.68,45
VCC  (via drill 0.3 pad 0.75, 0.4 pad 0.8)
  Top 0.2: IC3.6 v31.68,62.25 31.68,61.25 30.43,60 v26.43,60 IC3.1 | IC2.28 12.43,52.25 v12.68,52.5 | IC1.20 14.28,56.65 v14.18,56.75 | IC1.18 v14.18,58.25 | IC1.6 26.48,57.45 v26.43,57.5 | IC1.4 26.28,55.85 v26.43,55.75 | OP1.5 40.13,33.7 v40.43,33.75 | R5.2 45.18,27.25 v45.43,27 | R7.2 v45.43,24.75 | D1.A v33.43,71.5
  Top 0.6: BT1.11 35.53,95.85 35.93,96.25 37.68,96.25 v38.18,96.75 | v14.18,66.25 21.43,66.25 22.68,67.5 25.18,67.5 v25.43,67.75 25.68,67.5 v31.68,67.5 34.18,70 CP4.1 | X1.4 25.27,70.25 v25.43,70.25
  Top 0.8: v31.68,62.25 v42.43,62.25 | PAD4.1 v56.68,6
  Bottom 0.2: R2.5 37.26,86.92 37.18,87 37.18,87.85 | 37.18,87.85 37.18,88.7 | 37.18,88.7 37.18,89.25 37.51,89.57 | R2.8 37.51,89.57 | C8.2 36.93,91.9 37.18,91.65 37.18,89.9 37.51,89.57 | R2.7 37.23,88.65 37.18,88.7 | R2.6 37.18,87.85 | v40.43,33.75 45.18,33.75 45.43,33.5 | C9.2 v14.18,58.25 | v33.43,71.5 34.68,71.5 34.68,71.75 34.78,72 34.73,72.05
  Bottom 0.6: C6.2 31.68,63.25 | 49.68,1.87 49.66,1.84 | v12.68,52.5 C7.2 14.03,53.85 14.18,54 v14.18,56.75 v14.18,58.25 v14.18,66.25 | v26.43,55.75 v26.43,57.5 v26.43,60 | v25.43,70.25 v25.43,67.75 | v31.68,67.5 31.68,63.25 | v31.68,62.25 31.68,63.25
  Bottom 0.8: LED1.A 51.96,102.88 LED2.A LED3.A 35.78,100.42 | 35.78,100.42 35.26,100.23 LED4.A LED5.A LED6.A LED7.A LED8.A LED9.A LED10.A LED11.A LED12.A LED13.A LED14.A LED15.A LED16.A LED17.A LED18.A LED19.A LED20.A LED21.A LED22.A LED23.A 49.66,1.84 LED24.A 56.08,1.65 56.68,2.25 v56.68,5 v56.68,6 | 35.78,100.42 36.43,99.77 36.43,98.5 v38.18,96.75 35.68,94.25 C8.2 | v42.43,62.25 42.43,36.75 45.43,33.75 45.43,33.5 v45.43,27 v45.43,24.75 45.43,7.5 49.68,3.25 49.68,1.87 | S4.S1 34.73,72.05 35.18,72.5 37.68,72.5 40.18,70 CP4.1
XLAT  (via drill 0.3 pad 0.75)
  Top 0.2: IC2.26 11.68,51.25 12.93,50 v14.68,50 17.68,50 18.43,50.75 IC1.26 | 24.43,18.5 25.93,17 25.93,16 31.68,10.25 44.68,10.25 49.43,5.5 51.93,5.5 51.93,5.75 v52.18,6 | 24.43,18.5 23.43,18.5 17.43,24.5 17.43,26.25 v16.43,27.25 | CP7.1 v48.43,64 | v46.93,19 24.93,19 24.43,18.5 | 52.18,5.75 v52.18,6 | v52.18,6 PAD7.1
  Bottom 0.2: v14.68,50 14.68,29 v16.43,27.25 | v48.43,64 48.43,38.25 46.93,36.75 v46.93,19

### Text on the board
tPlace: ISP | SOUT | GND | BLANK | RST | VCC | SIN | VCC | SCK | MISO | MOSI | GND | SCLK | XLAT | + | - | BAT | + | - | CHARGE | DESIGN: THORSTEN MÜHLKE | DATE: 2012.05.25 | INSPIRED: NIKOLAI NIKITIN | LBB01v00 / LED BLINKY BALL
bPlace: BLANK | SIN | SOUT | BRIGHT | RESET | MODE | XLAT | GND | SCLK | VCC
